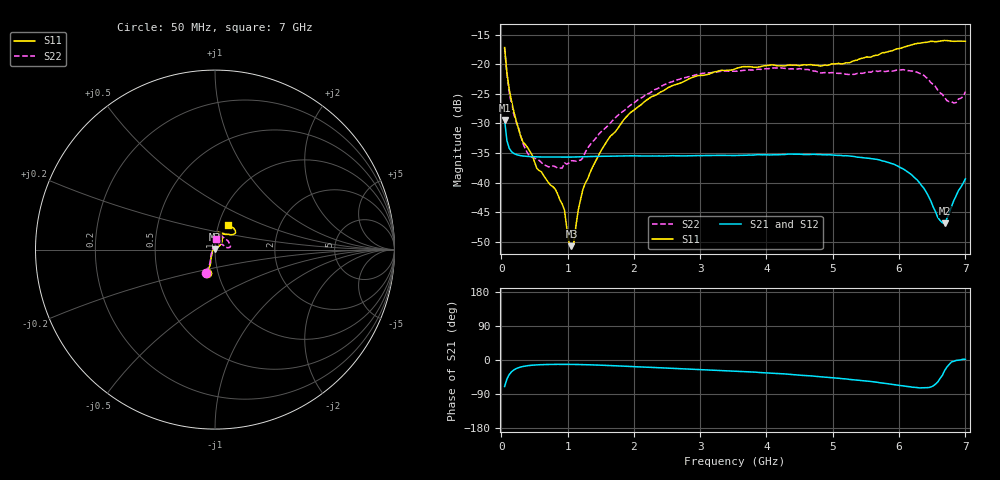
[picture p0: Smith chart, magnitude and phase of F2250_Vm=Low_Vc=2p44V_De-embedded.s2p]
! Integrated Device Technology
! Corporate Headquarters
! 6024 Silver Creek Valley Road
! San Jose, CA 95138  USA
! Phone:  1-408-284-8200
! Toll Free:  1-800-223-1366
! Webpage:  http://www.idt.com/
! Timing and RF Division
! 515 Groton Road, Suite 102
! Westford, MA 01886-6024
! Device:  F2250
! Description: Voltage Variable RF Attenuator
! Frequency:  50.0 -  6000.00 MHz
! Package:  3x3 mm Thin QFN Plastic Package: 16 pin
! Ports:  2 RF, 3 DC
!  Pin  1  = GND
!  Pin  2  = NC
!  Pin  3  = RF1  = Port 1
!  Pin  4  = NC
!  Pin  5  = GND
!  Pin  6  = GND
!  Pin  7  = GND
!  Pin  8  = GND
!  Pin  9  = NC
!  Pin 10  = RF2  = Port 2
!  Pin 11  = NC
!  Pin 12  = GND
!  Pin 13  = GND
!  Pin 14  = VCNTRL
!  Pin 15  = VDD
!  Pin 16  = VMODE
! Vcntrl:  2.440 Volts
! Vmode:  +0.000 Volts
! Vdd:  +3.30  Volts
! Current:  1.176 mA
! Data:  The device was measured on a the F2250 evaluation board which has
!  individual transmission lines to the RF pins.  Data was collected
!  using a calibrated network analyzer.  The evaluation board was
!  de-embedded using a TRL calibration technique.
!  The reference plane is the edge of the package pin.
! Misc:  SN 10
!  Action Tracker AT0258
! Date Measured:  2014-11-26
! Date:  2015-10-15  MJV
! Note:
!  Integrated Device Technology supplies this data as a sample of measured
!  data at the package pin for this product.  Your particular data for this
!  product may vary.
!  Data was taken at 25 degrees C.
!  Integrated Device Technology reserves the right to change this data at anytime.
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# GHz S dB R 50
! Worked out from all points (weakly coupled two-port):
!   201 points, 50 MHz to 7 GHz, reference 50 ohm
!   highest |S21| = -29.41 dB at 50 MHz (marker M1); lowest = -46.9 dB at 6.687 GHz (marker M2)
!   lowest |S11| = -50.7 dB at 1.058 GHz (marker M3), VSWR 1.01, Z = 49.8 + j0.244 ohm
!   |S11| at or under -10 dB: start of sweep to end of sweep
!   |S22| runs from -37.5 to -17.3 dB; largest |S21 - S12| = 6.2e-05
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0.05  -17.18 -108.7  -29.41 -69.8  -29.41 -69.8  -17.28 -111.0
0.08475  -21.44 -107.4  -32.92 -50.4  -32.92 -50.4  -21.75 -110.2
0.15425  -26.23 -116.6  -34.76 -31.2  -34.75 -31.2  -26.81 -122.4
0.29325  -32.20 -127.7  -35.43 -18.4  -35.43 -18.4  -32.10 -137.5
0.3975  -34.07 -141.6  -35.56 -15.0  -35.56 -15.0  -35.05 -160.5
0.5365  -37.60 -155.7  -35.63 -12.8  -35.63 -12.8  -36.03 178.0
0.91875  -43.60 158.3  -35.68 -11.5  -35.68 -11.5  -37.53 133.5
0.9535  -44.65 169.3  -35.68 -11.5  -35.68 -11.5  -36.65 131.2
1.023  -50.14 144.5  -35.67 -11.6  -35.67 -11.6  -36.64 116.0
1.05775  -50.71 122.7  -35.67 -11.6  -35.67 -11.6  -36.29 110.8
1.0925  -50.38 90.6  -35.66 -11.7  -35.65 -11.7  -36.30 106.2
1.162  -44.55 57.0  -35.64 -11.9  -35.64 -11.9  -36.23 95.5
1.2315  -41.11 44.1  -35.61 -12.1  -35.61 -12.1  -35.78 85.9
1.6485  -32.11 41.9  -35.52 -14.7  -35.52 -14.6  -29.87 64.6
2.37825  -24.87 47.3  -35.48 -20.3  -35.48 -20.3  -23.99 56.8
3.525  -20.80 72.4  -35.40 -29.5  -35.41 -29.5  -21.19 74.8
4.7065  -20.16 72.4  -35.20 -42.5  -35.20 -42.5  -21.15 72.3
5.85325  -17.81 40.5  -36.64 -63.3  -36.65 -63.3  -21.13 23.0
6.27025  -16.50 40.1  -39.50 -72.6  -39.51 -72.6  -21.35 9.7
6.68725  -15.99 48.8  -46.86 -27.7  -46.83 -27.3  -25.64 28.4
6.861  -16.13 55.1  -42.19 -1.2  -42.14 -1.2  -26.47 58.0
7  -16.13 63.2  -39.34 1.9  -39.31 1.8  -24.62 83.1
